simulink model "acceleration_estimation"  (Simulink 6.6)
settings: Solver=FixedStepDiscrete  StartTime=0.0  StopTime=1000.0  FixedStep=1  RelTol=1e-3
libraries: dspadpt3 x1

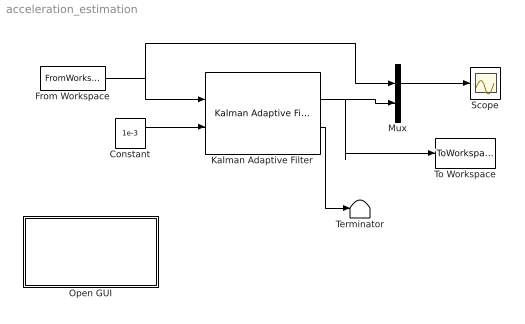
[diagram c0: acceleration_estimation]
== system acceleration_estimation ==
  Constant : Constant  Value=1e-3
  From Workspace : FromWorkspace  VariableName=[tout,x_accel]  SampleTime=1
  Kalman Adaptive Filter : dspadpt3/Kalman Adaptive Filter  SystemSampleTime=-1  Ntaps=50  Jmin=0.0077  q=0.01^2  ic0=0  K0=0.5  Adapt=off  RstPort=None
  Mux : Mux  Inputs=2
  Open GUI : Subsystem
  Scope : Scope
  Terminator : Terminator
  To Workspace : ToWorkspace  VariableName=simout  SampleTime=-1  SaveFormat=Array
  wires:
  From Workspace/1 -> Mux/1, Kalman Adaptive Filter/1
  Mux/1 -> Scope/1
  Kalman Adaptive Filter/1 -> Mux/2, To Workspace/1
  Constant/1 -> Kalman Adaptive Filter/2
  Kalman Adaptive Filter/2 -> Terminator/1

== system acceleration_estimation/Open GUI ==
